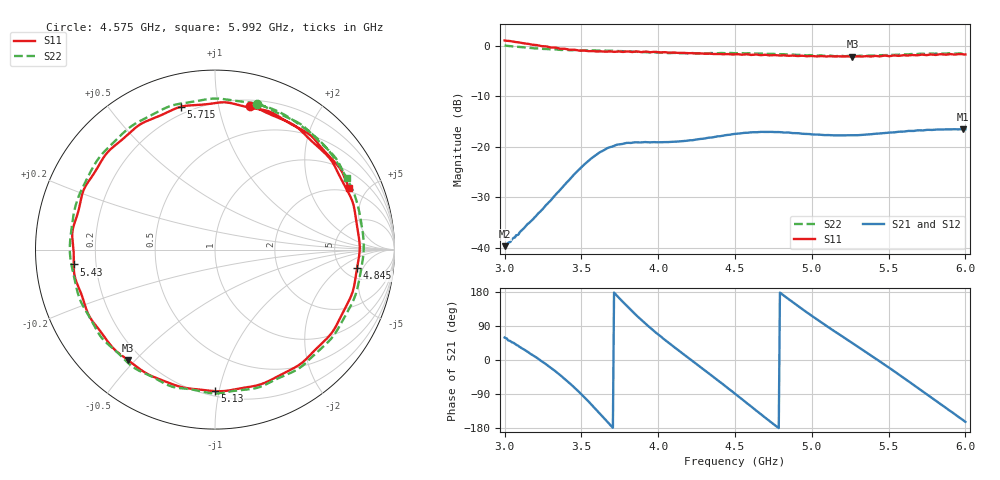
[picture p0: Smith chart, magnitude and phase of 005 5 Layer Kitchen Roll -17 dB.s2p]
!  04/11/2025  14:27:43
! Ref Plane: 0.000 mm
# MHZ S MA R  50
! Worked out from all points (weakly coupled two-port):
!   401 points, 3 GHz to 6 GHz, reference 50 ohm
!   highest |S21| = -16.48 dB at 5.985 GHz (marker M1); lowest = -39.6 dB at 3 GHz (marker M2)
!   lowest |S11| = -2.1 dB at 5.265 GHz (marker M3), VSWR 8.23, Z = 7.49 - j23.9 ohm
!   |S11| at or under -10 dB: nowhere
!   |S22| runs from -2.0 to 0.1 dB; largest |S21 - S12| = 0.0032
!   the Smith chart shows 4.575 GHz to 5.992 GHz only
!   S11 on the Smith chart (normalised r, x): 4.575 GHz: 0.25, +1.24; 4.845 GHz: 6.68, -3.83; 5.13 GHz: 0.23, -0.97; 5.43 GHz: 0.12, -0.05; 5.715 GHz: 0.16, +0.78; 5.992 GHz: 1.78, +3.77
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3000  1.132 -114.4  0.01043 59.4  0.01046 60.4  1.009 -116.9
3270  0.9888 177.8  0.02666 -11.2  0.02647 -9.7  0.932 175.3
3390  0.9376 140.1  0.04218 -49.3  0.04234 -48.6  0.9145 136.7
3502.5  0.9 97.4  0.06347 -91.6  0.06349 -91.0  0.9026 94.0
3607.5  0.8797 52.4  0.08611 -135.8  0.08631 -135.3  0.8968 50.2
3735  0.8797 -5.0  0.1056 168.0  0.1058 169.1  0.8899 -4.4
3862.5  0.8808 -57.4  0.1112 116.0  0.1119 117.3  0.8743 -55.0
4005  0.8627 -107.4  0.1113 66.1  0.1111 66.9  0.8552 -104.5
4245  0.8409 178.2  0.1181 -9.4  0.1185 -8.2  0.8438 179.6
4500  0.8261 99.7  0.1346 -89.2  0.1354 -88.3  0.8457 98.4
4575  0.8252 76.5  0.138 -113.1  0.1381 -112.4  0.8432 73.8
4717.5  0.8079 32.1  0.1409 -158.5  0.1411 -157.8  0.8346 28.6
4845  0.7982 -7.5  0.139 161.8  0.139 162.8  0.8208 -10.8
5002.5  0.7952 -54.0  0.1331 115.9  0.1331 116.7  0.8085 -56.7
5130  0.7886 -90.1  0.1305 80.8  0.1305 81.5  0.7992 -92.5
5265  0.7833 -128.1  0.1304 44.4  0.1307 45.1  0.7925 -129.7
5430  0.791 -174.0  0.1354 -0.2  0.1357 0.7  0.8056 -175.0
5505  0.7909 164.3  0.1386 -20.8  0.1392 -19.8  0.8132 164.2
5715  0.8186 103.5  0.1456 -80.8  0.1459 -79.7  0.8376 105.8
5985  0.8234 27.2  0.15 -158.6  0.1506 -157.7  0.8351 30.8
5992.5  0.8218 24.8  0.1498 -160.9  0.1502 -160.1  0.8334 28.4
6000  0.8223 22.3  0.1495 -163.2  0.1499 -162.4  0.8341 26.1
